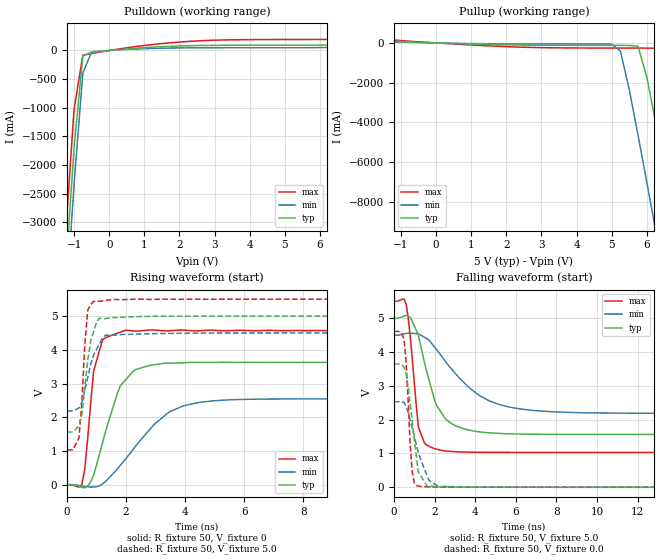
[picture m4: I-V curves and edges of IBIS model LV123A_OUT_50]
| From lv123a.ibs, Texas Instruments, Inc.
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|   Model LV123A_OUT_50
[Model]   LV123A_OUT_50
Model_type  Output
Polarity   Non-Inverting
Vmeas = 2.50v
Cref = 15pf
| variable   typ   min   max
C_comp   4.62pf   3.47pf   5.77pf
[Temperature Range]   25   85   -40
[Voltage Range]   5.0   4.5   5.5
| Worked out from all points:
|   slope of the pulldown table from 0 to 0.75 V, typ, clamps not added: 18.8 ohm
|   slope of the pullup table from 0 to 0.75 V, typ, clamps not added: 17.2 ohm
|   rising waveform, R_fixture 50, V_fixture 0: 20-80 % time 745ps typ, 1.55ns min, 343ps max; typ from 0 V to 3.63 V
|   falling waveform, R_fixture 50, V_fixture 5.0: 20-80 % time 1.02ns typ, 2.26ns min, 403ps max; typ from 5 V to 1.56 V
|   rising waveform, R_fixture 50, V_fixture 5.0: 20-80 % time 294ps typ, 452ps min, 192ps max; typ from 1.56 V to 5 V
|   falling waveform, R_fixture 50, V_fixture 0.0: 20-80 % time 432ps typ, 737ps min, 239ps max; typ from 3.64 V to 0 V
[Pulldown]
|   Voltage   I(typ)   I(min)   I(max)
-5V       -40.86A    -41.44A    -40.27A
-1.25V    -3.966A    -4.615A    -3.277A
-1V       -1.69A     -2.328A    -1.024A
-750mV    -95.47mA   -395.2mA   -80.63mA
-500mV    -31.61mA   -21.18mA   -52.4mA
1V        50.29mA    31.24mA    87.2mA
2.25V     83.32mA    46.61mA    158.1mA
3.25V     91.14mA    47.8mA     184mA
7V        108.5mA    62.97mA    205.8mA
8.25V     142.1mA    85.51mA    254.9mA
10V       202.1mA    122.1mA    356.9mA
[Pullup]
|   Voltage   I(typ)   I(min)   I(max)
-5V       343.1mA    193.8mA    632.1mA
1.25V     -68.16mA   -38.48mA   -126.3mA
5V        -123.3mA   -58.89mA   -259.3mA
5.25V     -123.4mA   -409.3mA   -259.4mA
5.75V     -164mA     -4.617A    -259.7mA
6V        -1.7A      -6.988A    -262.5mA
6.25V     -3.971A    -9.396A    -268.3mA
6.5V      -6.347A    -11.82A    -1.058A
6.75V     -8.763A    -14.27A    -3.287A
7.25V     -13.65A    -19.17A    -8.096A
7.5V      -16.1A     -21.64A    -10.54A
10V       -40.86A    -46.4A     -35.3A
[Ramp]
| variable   typ   min   max
dV/dt_r  2.1813E+00/7.3681E-10  1.5377E+00/1.5310E-09  2.7750E+00/3.0994E-10
dV/dt_f  2.1121E+00/9.8900E-10  1.4227E+00/2.2656E-09  2.7260E+00/4.2301E-10
R_load = 50
[Rising Waveform]
R_fixture = 50
V_fixture = 0
|   Time   V(typ)   V(min)   V(max)
0s        0V         0V         0V
500ps     -77.5mV    -42.1mV    430.1uV
600ps     -93.19mV   -54.38mV   464mV
900ps     288.1mV    -66.6mV    3.374V
1.2ns     1.236V     21.22mV    4.298V
1.8ns     2.93V      570.5mV    4.523V
2ns       3.128V     784.4mV    4.582V
3.4ns     3.604V     2.118V     4.561V
5ns       3.627V     2.491V     4.577V
25ns      3.627V     2.547V     4.571V
[Falling Waveform]
R_fixture = 50
V_fixture = 5.0
V_fixture_min = 4.5
V_fixture_max = 5.5
|   Time   V(typ)   V(min)   V(max)
0s        5V         4.5V       5.5V
600ps     5.079V     4.548V     5.415V
800ps     5.025V     4.556V     4.476V
1.2ns     4.5V       4.536V     1.791V
1.5ns     3.697V     4.437V     1.31V
2.1ns     2.421V     4.07V      1.124V
2.9ns     1.86V      3.45V      1.056V
4.2ns     1.64V      2.716V     1.034V
6.2ns     1.573V     2.318V     1.03V
25ns      1.562V     2.186V     1.03V
[Rising Waveform]
R_fixture = 50
V_fixture = 5.0
V_fixture_min = 4.5
V_fixture_max = 5.5
|   Time   V(typ)   V(min)   V(max)
0s        1.562V     2.186V     1.03V
400ps     1.739V     2.275V     1.383V
500ps     2.065V     2.434V     2.419V
600ps     2.88V      2.79V      4.16V
700ps     3.692V     3.177V     5.172V
900ps     4.541V     3.849V     5.437V
1.1ns     4.941V     4.183V     5.439V
1.3ns     4.927V     4.434V     5.463V
2.3ns     4.982V     4.464V     5.502V
25ns      5V         4.5V       5.5V
[Falling Waveform]
R_fixture = 50
V_fixture = 0.0
|   Time   V(typ)   V(min)   V(max)
0s        3.643V     2.525V     4.606V
500ps     3.544V     2.499V     4.357V
600ps     3.354V     2.392V     3.693V
800ps     2.468V     1.992V     1.24V
900ps     1.958V     1.756V     447.3mV
1ns       1.443V     1.512V     131.2mV
1.2ns     448.8mV    1.025V     35.77mV
1.7ns     -17.96mV   232.7mV    11.19mV
2.3ns     9.588mV    22.18mV    4.676mV
25ns      0V         0V         7.013uV
